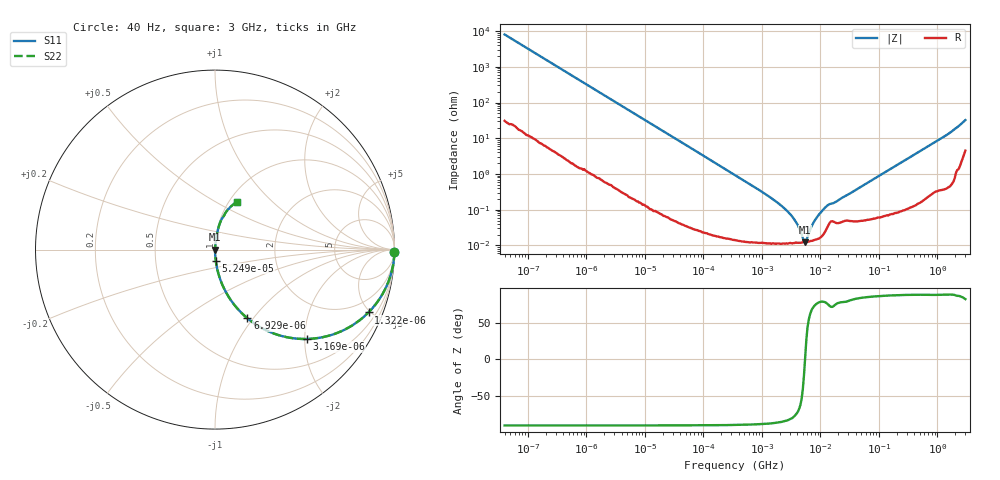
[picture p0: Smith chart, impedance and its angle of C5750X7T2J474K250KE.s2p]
! S-parameter Generated by TDK Corporation
! Copyright(C) 2015 TDK Corporation.
! All Rights Reserved.
! TDK P/N: C5750X7T2J474K250KE (Multilayer Ceramic Chip Capacitors)
! Property: C=470nF
! Size(LxWxT): 5.7x5x2.5mm, 0.224x0.197x0.098inches
! Model Type: s2p (Touchstone File Format Version 1.0)
! Frequency: DC=Yes Start=0.00004MHz Stop=3000MHz 396points Log-sweep
! Note: This model was converted from impedance.
! Model Generated on Jun. 23, 2015
! Hash(MD5):
! Port Assignments:
!  1 ---| |--- 2
! Applicable Conditions:
!  Temperature = 25 degC
!  DC Bias Voltage = 0 V
!  Small Signal Operation
! Terms and conditions regarding TDK Simulation Models
! (1)This simulation model is being provided solely for informational purposes. Please refer to the specifications of the products in terms of detailed characteristics of such products.
! (2)In no event shall TDK Corporation of any of its subsidiaries be liable for any loss or damage arising, directly or indirectly,
!  From any information contained in this simulation model, including, but not limited to loss or damages arising from any inaccuracies, omissions or errors in connection with such information.
! (3)Any and all copyrights on this simulation model are owned by TDK Corporation.
!  Duplication or redistribution of this simulation model without prior written permission from TDK Corporation is prohibited.
! (4)This simulation model is subject to any modification or change without any prior notice.
! (5)Neither TDK Corporation nor any of its subsidiaries shall make any warranty, express or implied,
!  Including but not limited to the correctness, implied warranties of merchantability and fitness for a particular purpose with respect to this simulation models.
! (6)The use of this simulation model shall be deemed to have consented to the terms and conditions hereof.
# MHz S MA R 50
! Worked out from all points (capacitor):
!   395 points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, 40 Hz to 3 GHz, reference 50 ohm
!   read as one part in series: C = 497 nF near 41.88 Hz
!   lowest |Z| = 12.4 mohm at 5.481 MHz (marker M1)
!   series resonance near 5.457 MHz, so ESL is about 1.7 nH
!   S11 on the Smith chart (normalised r, x): 40 Hz: open; 1.322 kHz: 1.02, -4.88; 3.169 kHz: 1.01, -2.04; 6.929 kHz: 1.00, -0.93; 52.49 kHz: 1.00, -0.12; 3 GHz: 1.09, +0.64
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4e-05  0.9999 -0.7  0.01245 89.1  0.01245 89.1  0.9999 -0.7
0.0002520917  0.9967 -4.5  0.07818 85.3  0.07818 85.3  0.9967 -4.5
0.000834128  0.9672 -14.5  0.2504 75.3  0.2504 75.3  0.9672 -14.5
0.001321622  0.9241 -22.2  0.3786 67.5  0.3786 67.5  0.9241 -22.2
0.003168613  0.7127 -44.3  0.6988 45.5  0.6988 45.5  0.7127 -44.3
0.006928769  0.4227 -64.8  0.9046 25.0  0.9046 25.0  0.4227 -64.8
0.01739424  0.1832 -79.2  0.9823 10.6  0.9823 10.6  0.1832 -79.2
0.05249338  0.06187 -86.1  0.9977 3.5  0.9977 3.5  0.06187 -86.1
0.3464102  0.009407 -88.6  0.9998 0.5  0.9998 0.5  0.009407 -88.6
1.315913  0.002354 -87.1  0.9999 0.1  0.9999 0.1  0.002354 -87.1
2.624455  0.0009663 -83.1  0.9999 0.1  0.9999 0.1  0.0009663 -83.1
3.971241  0.0004065 -73.0  0.9999 0.0  0.9999 0.0  0.0004065 -73.0
5.234209  0.0001341 -21.1  0.9999 0.0  0.9999 0.0  0.0001341 -21.1
5.480732  0.0001239 2.4  0.9999 -0.0  0.9999 -0.0  0.0001239 2.4
7.22376  0.0003711 68.7  0.9999 -0.0  0.9999 -0.0  0.0003711 68.7
9.521122  0.0007467 77.8  0.9998 -0.0  0.9998 -0.0  0.0007467 77.8
13.75903  0.001386 74.1  0.9996 -0.1  0.9996 -0.1  0.001386 74.1
18.13479  0.001645 74.6  0.9996 -0.1  0.9996 -0.1  0.001645 74.6
150.6385  0.01326 86.1  0.9992 -0.8  0.9992 -0.8  0.01326 86.1
1040.901  0.088 82.8  0.9928 -5.0  0.9928 -5.0  0.088 82.8
1893.418  0.1679 78.2  0.9796 -9.7  0.9796 -9.7  0.1679 78.2
3000  0.2953 65.0  0.9151 -17.0  0.9151 -17.0  0.2953 65.0
